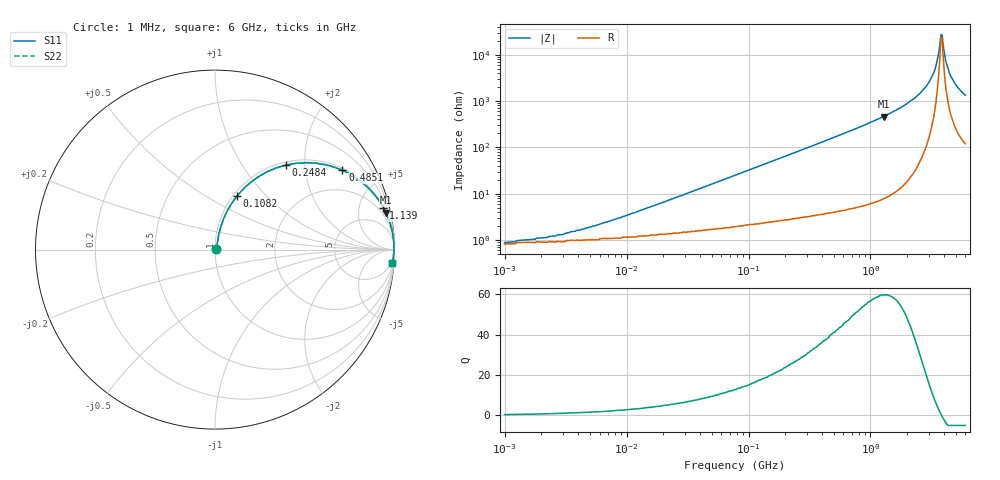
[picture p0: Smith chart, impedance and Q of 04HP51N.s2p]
# MHz S MA R 50
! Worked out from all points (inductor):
!   378 points, 1 MHz to 6 GHz, reference 50 ohm
!   read as one part in series: L = 51.2 nH near 11.02 MHz
!   highest Q = 59.8 at 1.279 GHz (marker M1), where L = 57.5 nH
!   self-resonance near 3.782 GHz
!   S11 on the Smith chart (normalised r, x): 1 MHz: 1.02, +0.01; 108.2 MHz: 1.04, +0.69; 248.4 MHz: 1.06, +1.60; 485.1 MHz: 1.08, +3.16; 1.139 GHz: 1.15, +8.01; 6 GHz: 3, -26
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1  0.008925 20.7  0.992 -0.2  0.992 -0.2  0.008925 20.7
2.243  0.011 37.9  0.991 -0.4  0.991 -0.4  0.011 37.9
4.279  0.017 53.3  0.99 -0.8  0.99 -0.8  0.017 53.3
18.312  0.059 74.2  0.985 -3.3  0.985 -3.3  0.059 74.2
78.359  0.24 71.7  0.952 -13.8  0.952 -13.8  0.24 71.7
108.24  0.322 67.7  0.927 -18.8  0.927 -18.8  0.322 67.7
248.409  0.614 50.1  0.767 -37.8  0.767 -37.8  0.614 50.1
335.312  0.724 41.9  0.668 -46.3  0.668 -46.3  0.724 41.9
485.059  0.836 31.9  0.529 -56.7  0.529 -56.7  0.836 31.9
1139.186  0.966 14.0  0.241 -75.1  0.241 -75.1  0.966 14.0
1278.506  0.974 12.2  0.211 -76.9  0.211 -76.9  0.974 12.2
1434.864  0.98 10.5  0.183 -78.5  0.183 -78.5  0.98 10.5
2276.372  0.994 5.0  0.088 -83.5  0.088 -83.5  0.994 5.0
2934.141  0.997 2.5  0.044 -84.3  0.044 -84.3  0.997 2.5
3448.517  0.997 1.0  0.017 -79.5  0.017 -79.5  0.997 1.0
3611.4  0.997 0.5  0.009775 -71.6  0.009775 -71.6  0.997 0.5
3781.976  0.997 0.1  0.003659 -29.3  0.003659 -29.3  0.997 0.1
3870.263  0.997 -0.1  0.003827 30.6  0.003827 30.6  0.997 -0.1
4147.681  0.996 -0.8  0.014 73.8  0.014 73.8  0.996 -0.8
4444.984  0.996 -1.4  0.025 79.2  0.025 79.2  0.996 -1.4
5105.049  0.994 -2.7  0.048 81.1  0.048 81.1  0.994 -2.7
6000  0.99 -4.3  0.075 80.5  0.075 80.5  0.99 -4.3
